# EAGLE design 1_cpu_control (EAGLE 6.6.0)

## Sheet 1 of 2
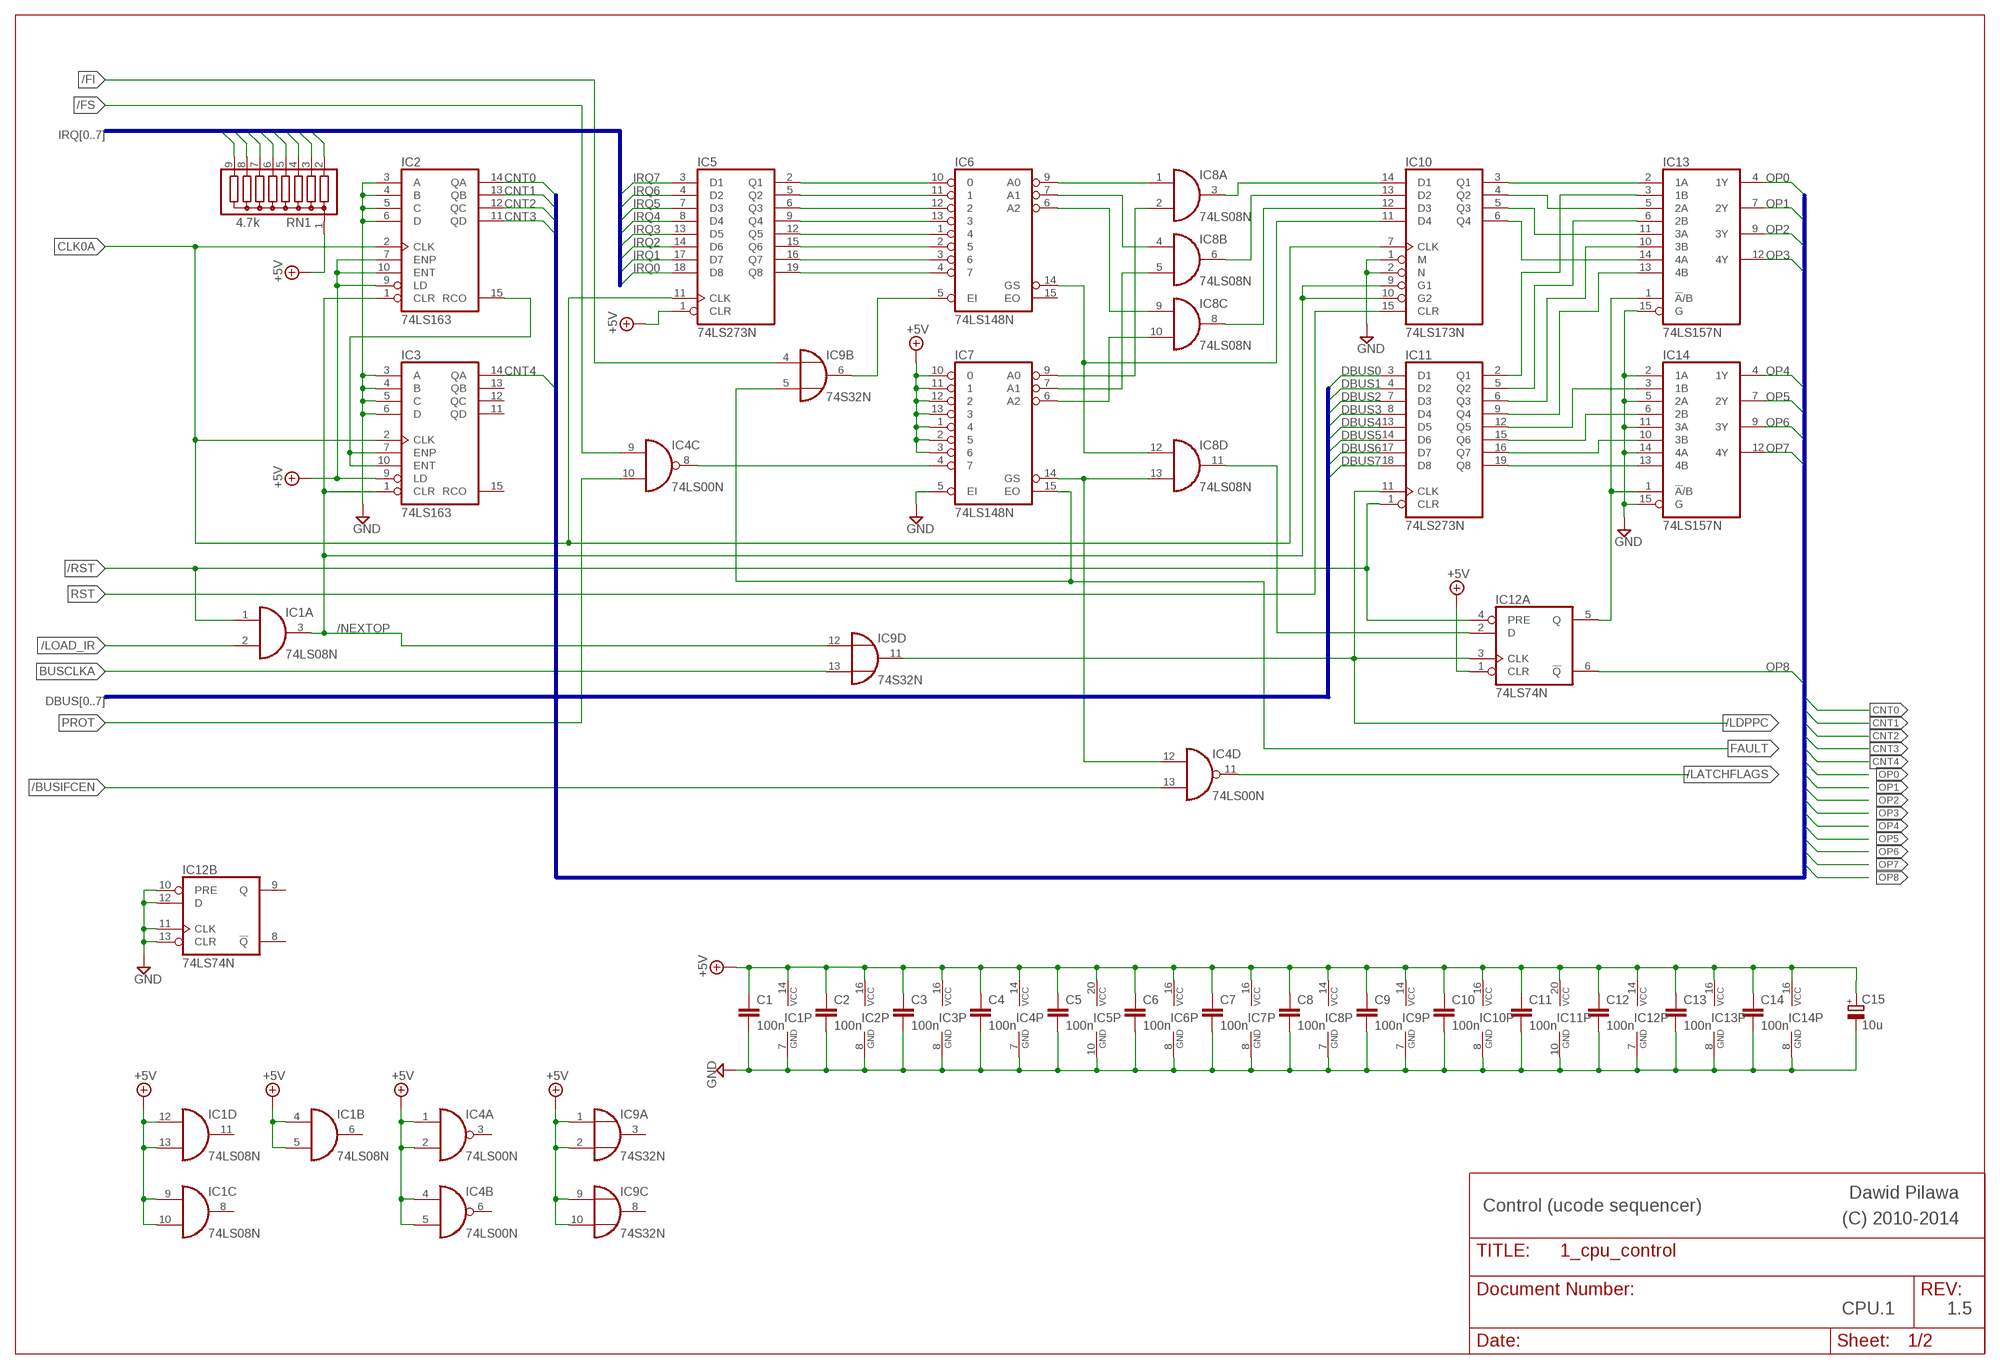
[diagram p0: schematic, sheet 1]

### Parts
C1  100n  C-EU050-024X044  [C050-024X044]
C2  100n  C-EU050-024X044  [C050-024X044]
C3  100n  C-EU050-024X044  [C050-024X044]
C4  100n  C-EU050-024X044  [C050-024X044]
C5  100n  C-EU050-024X044  [C050-024X044]
C6  100n  C-EU050-024X044  [C050-024X044]
C7  100n  C-EU050-024X044  [C050-024X044]
C8  100n  C-EU050-024X044  [C050-024X044]
C9  100n  C-EU050-024X044  [C050-024X044]
C10  100n  C-EU050-024X044  [C050-024X044]
C11  100n  C-EU050-024X044  [C050-024X044]
C12  100n  C-EU050-024X044  [C050-024X044]
C13  100n  C-EU050-024X044  [C050-024X044]
C14  100n  C-EU050-024X044  [C050-024X044]
C15  10u  CPOL-EUE5-6  [E5-6]
IC1  74LS08N  [DIL14]
IC2  74LS163  74160N  [DIL16]
IC3  74LS163  74160N  [DIL16]
IC4  74LS00N  [DIL14]
IC5  74LS273N  74273N  [DIL20]
IC6  74LS148N  [DIL16]
IC7  74LS148N  [DIL16]
IC8  74LS08N  [DIL14]
IC9  74S32N  [DIL14]
IC10  74LS173N  [DIL16]
IC11  74LS273N  74273N  [DIL20]
IC12  74LS74N  [DIL14]
IC13  74LS157N  [DIL16]
IC14  74LS157N  [DIL16]
RN1  4.7k  G08R  [SIL9]

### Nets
+5V: C1.1 C2.1 C3.1 C4.1 C5.1 C6.1 C7.1 C8.1 C9.1 C10.1 C11.1 C12.1 C13.1 C14.1 C15.+ IC1.4(B:I0) IC1.5(B:I1) IC1.9(C:I0) IC1.10(C:I1) IC1.12(D:I0) IC1.13(D:I1) IC1.14(P:VCC) IC2.7(ENP) IC2.9(LD) IC2.10(ENT) IC2.16(VCC) IC3.9(LD) IC3.16(VCC) IC4.1(A:I0) IC4.2(A:I1) IC4.4(B:I0) IC4.5(B:I1) IC4.14(P:VCC) IC5.1(CLR) IC5.20(VCC) IC6.16(VCC) IC7.1 IC7.2 IC7.3 IC7.10 IC7.11 IC7.12 IC7.13 IC7.16(VCC) IC8.14(P:VCC) IC9.1(A:I0) IC9.2(A:I1) IC9.9(C:I0) IC9.10(C:I1) IC9.14(P:VCC) IC10.16(VCC) IC11.20(VCC) IC12.1(A:CLR) IC12.14(P:VCC) IC13.16(VCC) IC14.16(VCC) RN1.1 ; also sheet 2
/BUSIFCEN: IC4.13(D:I1) ; also sheet 2
/FAULT_PF: IC4.8(C:O) IC7.4
/FI: IC9.4(B:I0) ; also sheet 2
/FS: IC4.9(C:I0) ; also sheet 2
/LATCHFLAGS: IC4.11(D:O) ; also sheet 2
/LDPPC: IC9.11(D:O) IC11.11(CLK) IC12.3(A:CLK) ; also sheet 2
/LOAD_IR: IC1.2(A:I1) ; also sheet 2
/NEXTOP: IC1.3(A:O) IC2.1(CLR) IC3.1(CLR) IC9.12(D:I0) IC10.9(G1) IC10.10(G2)
/RST: IC1.1(A:I0) IC11.1(CLR) IC12.4(A:PRE) ; also sheet 2
BUSCLKA: IC9.13(D:I1) ; also sheet 2
CLK0A: IC2.2(CLK) IC3.2(CLK) IC5.11(CLK) IC10.7(CLK) ; also sheet 2
CNT0: IC2.14(QA) ; also sheet 2
CNT1: IC2.13(QB) ; also sheet 2
CNT2: IC2.12(QC) ; also sheet 2
CNT3: IC2.11(QD) ; also sheet 2
CNT4: IC3.14(QA) ; also sheet 2
DBUS0: IC11.3(D1) ; also sheet 2
DBUS1: IC11.4(D2) ; also sheet 2
DBUS2: IC11.7(D3) ; also sheet 2
DBUS3: IC11.8(D4) ; also sheet 2
DBUS4: IC11.13(D5) ; also sheet 2
DBUS5: IC11.14(D6) ; also sheet 2
DBUS6: IC11.17(D7) ; also sheet 2
DBUS7: IC11.18(D8) ; also sheet 2
FAULT: IC7.15(EO) IC9.5(B:I1) ; also sheet 2
GND: C1.2 C2.2 C3.2 C4.2 C5.2 C6.2 C7.2 C8.2 C9.2 C10.2 C11.2 C12.2 C13.2 C14.2 C15.- IC1.7(P:GND) IC2.3(A) IC2.4(B) IC2.5(C) IC2.6(D) IC2.8(GND) IC3.3(A) IC3.4(B) IC3.5(C) IC3.6(D) IC3.8(GND) IC4.7(P:GND) IC5.10(GND) IC6.8(GND) IC7.5(EI) IC7.8(GND) IC8.7(P:GND) IC9.7(P:GND) IC10.1(M) IC10.2(N) IC10.8(GND) IC11.10(GND) IC12.7(P:GND) IC12.10(B:PRE) IC12.11(B:CLK) IC12.12(B:D) IC12.13(B:CLR) IC13.8(GND) IC13.15(G) IC14.2(1A) IC14.5(2A) IC14.8(GND) IC14.11(3A) IC14.14(4A) IC14.15(G) ; also sheet 2
IRQ0: IC5.18(D8) RN1.9 ; also sheet 2
IRQ1: IC5.17(D7) RN1.8 ; also sheet 2
IRQ2: IC5.14(D6) RN1.7 ; also sheet 2
IRQ3: IC5.13(D5) RN1.6 ; also sheet 2
IRQ4: IC5.8(D4) RN1.5 ; also sheet 2
IRQ5: IC5.7(D3) RN1.4 ; also sheet 2
IRQ6: IC5.4(D2) RN1.3 ; also sheet 2
IRQ7: IC5.3(D1) RN1.2 ; also sheet 2
N$1: IC6.9(A0) IC8.1(A:I0)
N$2: IC2.15(RCO) IC3.7(ENP) IC3.10(ENT)
N$3: IC7.9(A0) IC8.2(A:I1)
N$4: IC6.7(A1) IC8.4(B:I0)
N$5: IC7.7(A1) IC8.5(B:I1)
N$6: IC7.6(A2) IC8.10(C:I1)
N$7: IC6.6(A2) IC8.9(C:I0)
N$9: IC6.14(GS) IC8.12(D:I0) IC10.11(D4)
N$10: IC4.12(D:I0) IC7.14(GS) IC8.13(D:I1)
N$11: IC8.3(A:O) IC10.14(D1)
N$12: IC8.6(B:O) IC10.13(D2)
N$13: IC8.8(C:O) IC10.12(D3)
N$14: IC8.11(D:O) IC12.2(A:D)
N$16: IC11.5(Q2) IC13.6(2B)
N$18: IC10.3(Q1) IC13.2(1A)
N$19: IC10.4(Q2) IC13.5(2A)
N$20: IC10.5(Q3) IC13.11(3A)
N$21: IC10.6(Q4) IC13.14(4A)
N$22: IC11.19(Q8) IC14.13(4B)
N$23: IC11.16(Q7) IC14.10(3B)
N$24: IC11.15(Q6) IC14.6(2B)
N$25: IC11.12(Q5) IC14.3(1B)
N$26: IC11.2(Q1) IC13.3(1B)
N$27: IC6.5(EI) IC9.6(B:O)
N$28: IC11.6(Q3) IC13.10(3B)
N$30: IC11.9(Q4) IC13.13(4B)
N$47: IC12.5(A:Q) IC13.1(!A!/B) IC14.1(!A!/B)
N$57: IC5.19(Q8) IC6.4
N$58: IC5.16(Q7) IC6.3
N$59: IC5.15(Q6) IC6.2
N$60: IC5.12(Q5) IC6.1
N$61: IC5.9(Q4) IC6.13
N$62: IC5.6(Q3) IC6.12
N$63: IC5.5(Q2) IC6.11
N$64: IC5.2(Q1) IC6.10
OP0: IC13.4(1Y) ; also sheet 2
OP1: IC13.7(2Y) ; also sheet 2
OP2: IC13.9(3Y) ; also sheet 2
OP3: IC13.12(4Y) ; also sheet 2
OP4: IC14.4(1Y) ; also sheet 2
OP5: IC14.7(2Y) ; also sheet 2
OP6: IC14.9(3Y) ; also sheet 2
OP7: IC14.12(4Y) ; also sheet 2
OP8: IC12.6(A:!Q) ; also sheet 2
PROT: IC4.10(C:I1) ; also sheet 2
RST: IC10.15(CLR) ; also sheet 2
Unconnected: IC1.6(B:O) IC1.8(C:O) IC1.11(D:O) IC3.11(QD) IC3.12(QC) IC3.13(QB) IC3.15(RCO) IC4.3(A:O) IC4.6(B:O) IC6.15(EO) IC9.3(A:O) IC9.8(C:O) IC12.8(B:!Q) IC12.9(B:Q)

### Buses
DBUS[0..7]
UCADR:OP[0..8],CNT[0..4]
IRQ[0..7]

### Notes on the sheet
- Dawid Pilawa
- Control (ucode sequencer) | (C) 2010-2014
- CPU.1 | 1.5

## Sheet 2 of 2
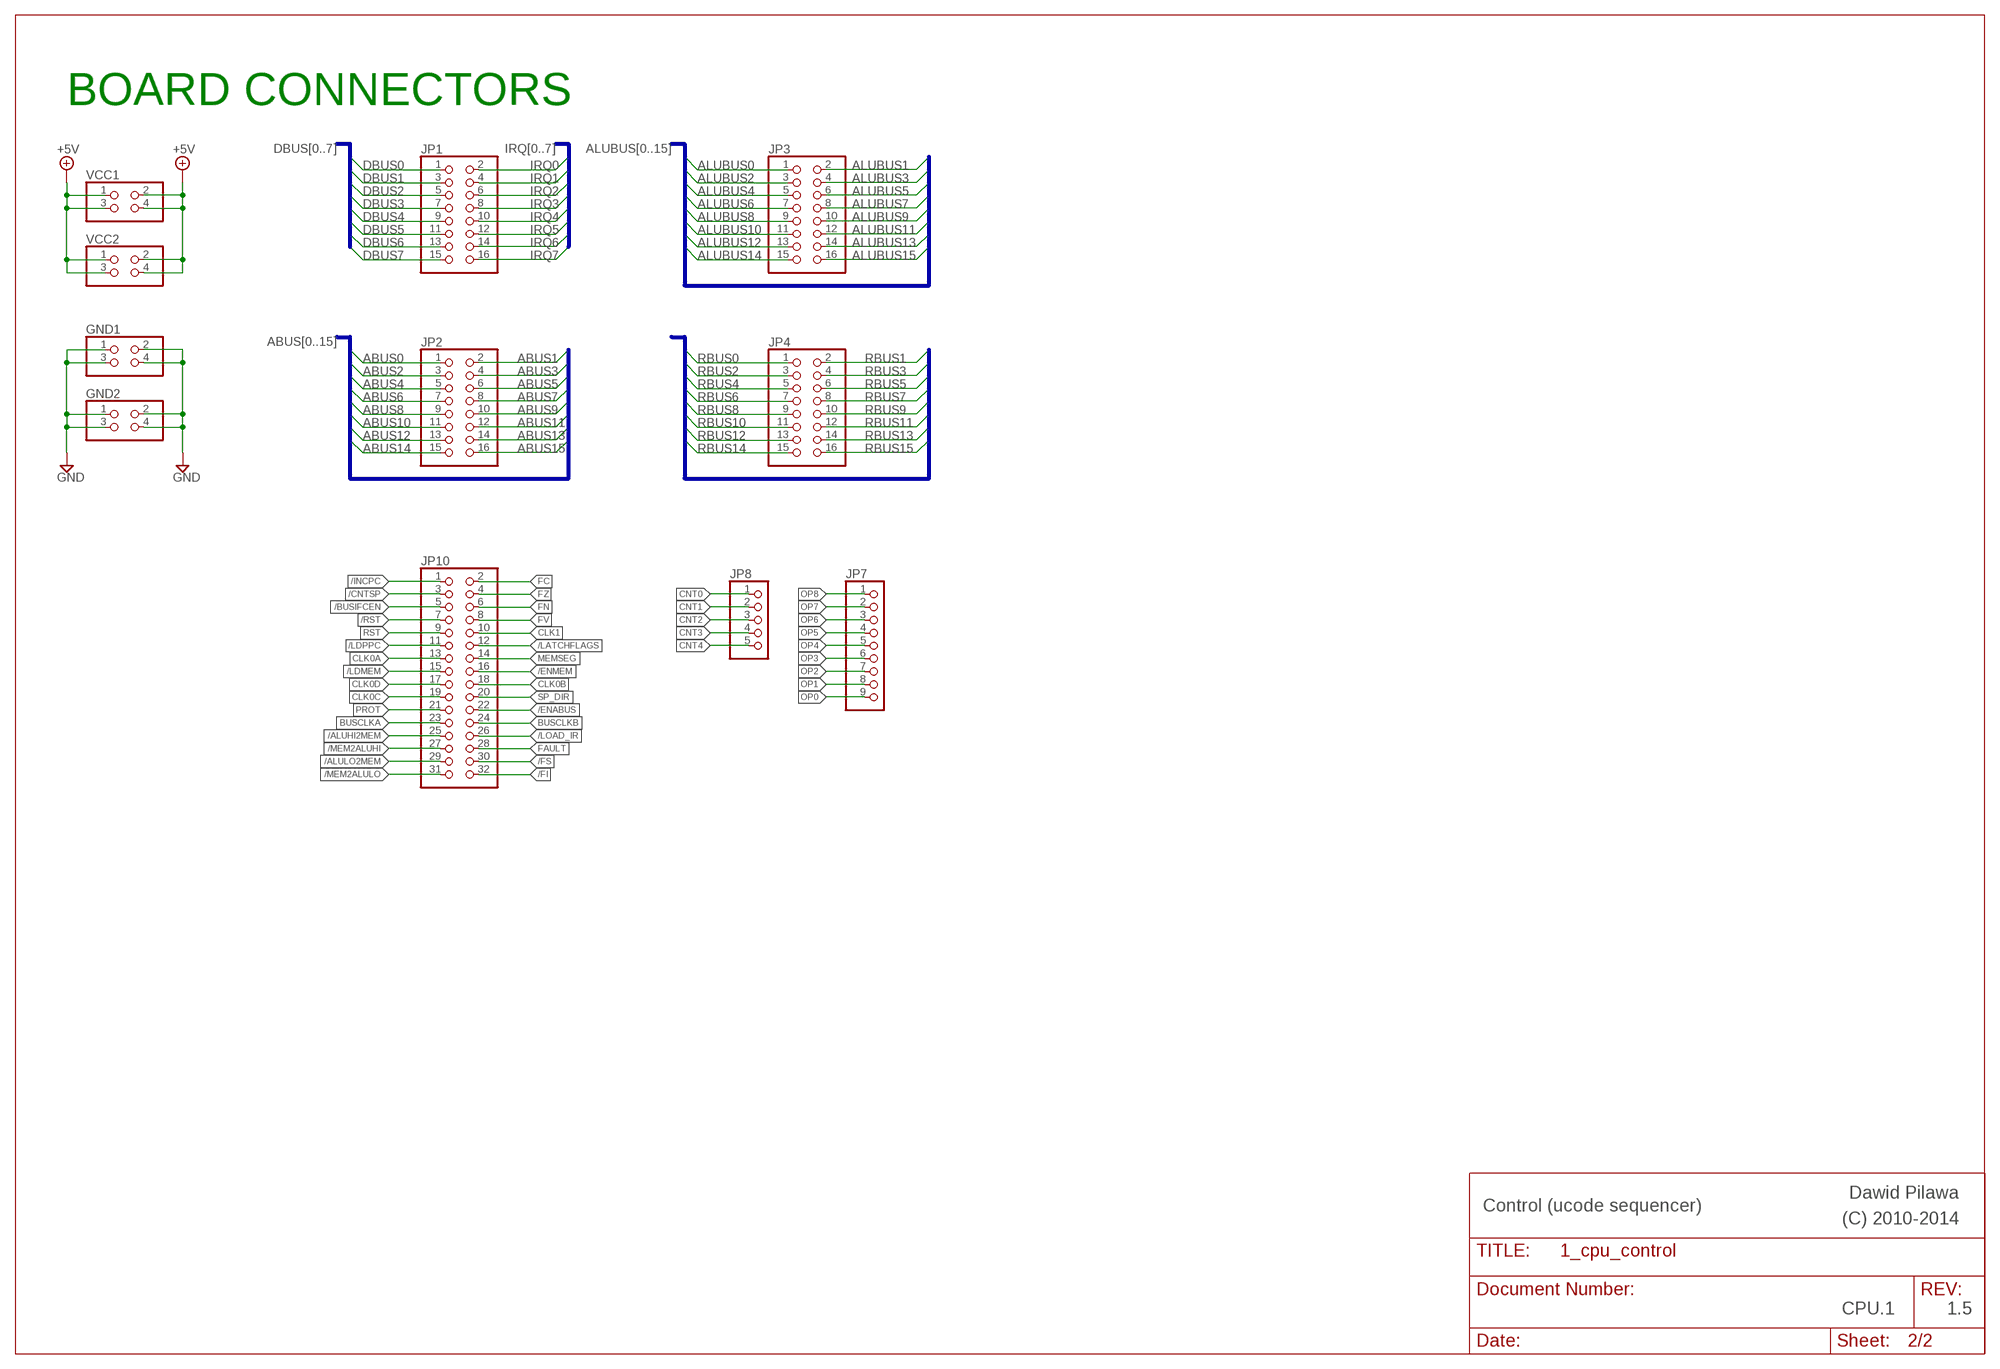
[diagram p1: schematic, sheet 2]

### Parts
GND1  PINHD-2X2  [2X02]
GND2  PINHD-2X2  [2X02]
JP1  PINHD-2X8  [2X08]
JP2  PINHD-2X8  [2X08]
JP3  PINHD-2X8  [2X08]
JP4  PINHD-2X8  [2X08]
JP7  PINHD-1X9  [1X09]
JP8  PINHD-1X5  [1X05]
JP10  PINHD-2X16  [2X16]
VCC1  PINHD-2X2  [2X02]
VCC2  PINHD-2X2  [2X02]

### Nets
+5V: VCC1.1 VCC1.2 VCC1.3 VCC1.4 VCC2.1 VCC2.2 VCC2.3 VCC2.4 ; also sheet 1
/ALUHI2MEM: JP10.25
/ALULO2MEM: JP10.29
/BUSIFCEN: JP10.5 ; also sheet 1
/CNTSP: JP10.3
/ENABUS: JP10.22
/ENMEM: JP10.16
/FI: JP10.32 ; also sheet 1
/FS: JP10.30 ; also sheet 1
/INCPC: JP10.1
/LATCHFLAGS: JP10.12 ; also sheet 1
/LDMEM: JP10.15
/LDPPC: JP10.11 ; also sheet 1
/LOAD_IR: JP10.26 ; also sheet 1
/MEM2ALUHI: JP10.27
/MEM2ALULO: JP10.31
/RST: JP10.7 ; also sheet 1
ABUS0: JP2.1
ABUS1: JP2.2
ABUS2: JP2.3
ABUS3: JP2.4
ABUS4: JP2.5
ABUS5: JP2.6
ABUS6: JP2.7
ABUS7: JP2.8
ABUS8: JP2.9
ABUS9: JP2.10
ABUS10: JP2.11
ABUS11: JP2.12
ABUS12: JP2.13
ABUS13: JP2.14
ABUS14: JP2.15
ABUS15: JP2.16
ALUBUS0: JP3.1
ALUBUS1: JP3.2
ALUBUS2: JP3.3
ALUBUS3: JP3.4
ALUBUS4: JP3.5
ALUBUS5: JP3.6
ALUBUS6: JP3.7
ALUBUS7: JP3.8
ALUBUS8: JP3.9
ALUBUS9: JP3.10
ALUBUS10: JP3.11
ALUBUS11: JP3.12
ALUBUS12: JP3.13
ALUBUS13: JP3.14
ALUBUS14: JP3.15
ALUBUS15: JP3.16
BUSCLKA: JP10.23 ; also sheet 1
BUSCLKB: JP10.24
CLK0A: JP10.13 ; also sheet 1
CLK0B: JP10.18
CLK0C: JP10.19
CLK0D: JP10.17
CLK1: JP10.10
CNT0: JP8.1 ; also sheet 1
CNT1: JP8.2 ; also sheet 1
CNT2: JP8.3 ; also sheet 1
CNT3: JP8.4 ; also sheet 1
CNT4: JP8.5 ; also sheet 1
DBUS0: JP1.1 ; also sheet 1
DBUS1: JP1.3 ; also sheet 1
DBUS2: JP1.5 ; also sheet 1
DBUS3: JP1.7 ; also sheet 1
DBUS4: JP1.9 ; also sheet 1
DBUS5: JP1.11 ; also sheet 1
DBUS6: JP1.13 ; also sheet 1
DBUS7: JP1.15 ; also sheet 1
FAULT: JP10.28 ; also sheet 1
FC: JP10.2
FN: JP10.6
FV: JP10.8
FZ: JP10.4
GND: GND1.1 GND1.2 GND1.3 GND1.4 GND2.1 GND2.2 GND2.3 GND2.4 ; also sheet 1
IRQ0: JP1.2 ; also sheet 1
IRQ1: JP1.4 ; also sheet 1
IRQ2: JP1.6 ; also sheet 1
IRQ3: JP1.8 ; also sheet 1
IRQ4: JP1.10 ; also sheet 1
IRQ5: JP1.12 ; also sheet 1
IRQ6: JP1.14 ; also sheet 1
IRQ7: JP1.16 ; also sheet 1
MEMSEG: JP10.14
OP0: JP7.9 ; also sheet 1
OP1: JP7.8 ; also sheet 1
OP2: JP7.7 ; also sheet 1
OP3: JP7.6 ; also sheet 1
OP4: JP7.5 ; also sheet 1
OP5: JP7.4 ; also sheet 1
OP6: JP7.3 ; also sheet 1
OP7: JP7.2 ; also sheet 1
OP8: JP7.1 ; also sheet 1
PROT: JP10.21 ; also sheet 1
RBUS0: JP4.1
RBUS1: JP4.2
RBUS2: JP4.3
RBUS3: JP4.4
RBUS4: JP4.5
RBUS5: JP4.6
RBUS6: JP4.7
RBUS7: JP4.8
RBUS8: JP4.9
RBUS9: JP4.10
RBUS10: JP4.11
RBUS11: JP4.12
RBUS12: JP4.13
RBUS13: JP4.14
RBUS14: JP4.15
RBUS15: JP4.16
RST: JP10.9 ; also sheet 1
SP_DIR: JP10.20

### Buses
DBUS[0..7]
IRQ[0..7]
ALUBUS[0..15]
RBUS[0..15]
ABUS[0..15]

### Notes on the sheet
- BOARD CONNECTORS
- Dawid Pilawa
- Control (ucode sequencer) | (C) 2010-2014
- CPU.1 | 1.5

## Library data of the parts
C1-C14 = rcl:C-EU: CAPACITOR, European symbol
C15 = rcl:CPOL-EU: POLARIZED CAPACITOR, European symbol
GND1 GND2 VCC1 VCC2 = pinhead:PINHD-2X2: PIN HEADER
IC1 IC8 = 74xx-eu:74*08: Quad 2-input AND gate
IC2 IC3 = 74xx-eu:74*160: Synchronous 4-bit COUNTER
IC4 = 74xx-eu:74*00: Quad 2-input NAND gate
IC5 IC11 = 74xx-eu:74*273: Octal D type FLIP FLOP, clear
IC6 IC7 = 74xx-eu:74*148: 10-line to 4-line and 8-line to 3-line PRIORITY ENCODER
IC9 = 74xx-eu:74*32: Quad 2-input OR gate
IC10 = 74xx-eu:74*173: 4-bit D type REGISTER, 3-state
IC12 = 74xx-eu:74*74: Dual D type positive edge triggered FLIP FLOP, preset and clear
IC13 IC14 = 74xx-eu:74*157: Quadruple 2-line to 1-line data SELECTOR/MULTIPLEXER
JP1-JP4 = pinhead:PINHD-2X8: PIN HEADER
JP7 = pinhead:PINHD-1X9: PIN HEADER
JP8 = pinhead:PINHD-1X5: PIN HEADER
JP10 = pinhead:PINHD-2X16: PIN HEADER
RN1 = resistor-sil:G08R: SIL RESISTOR

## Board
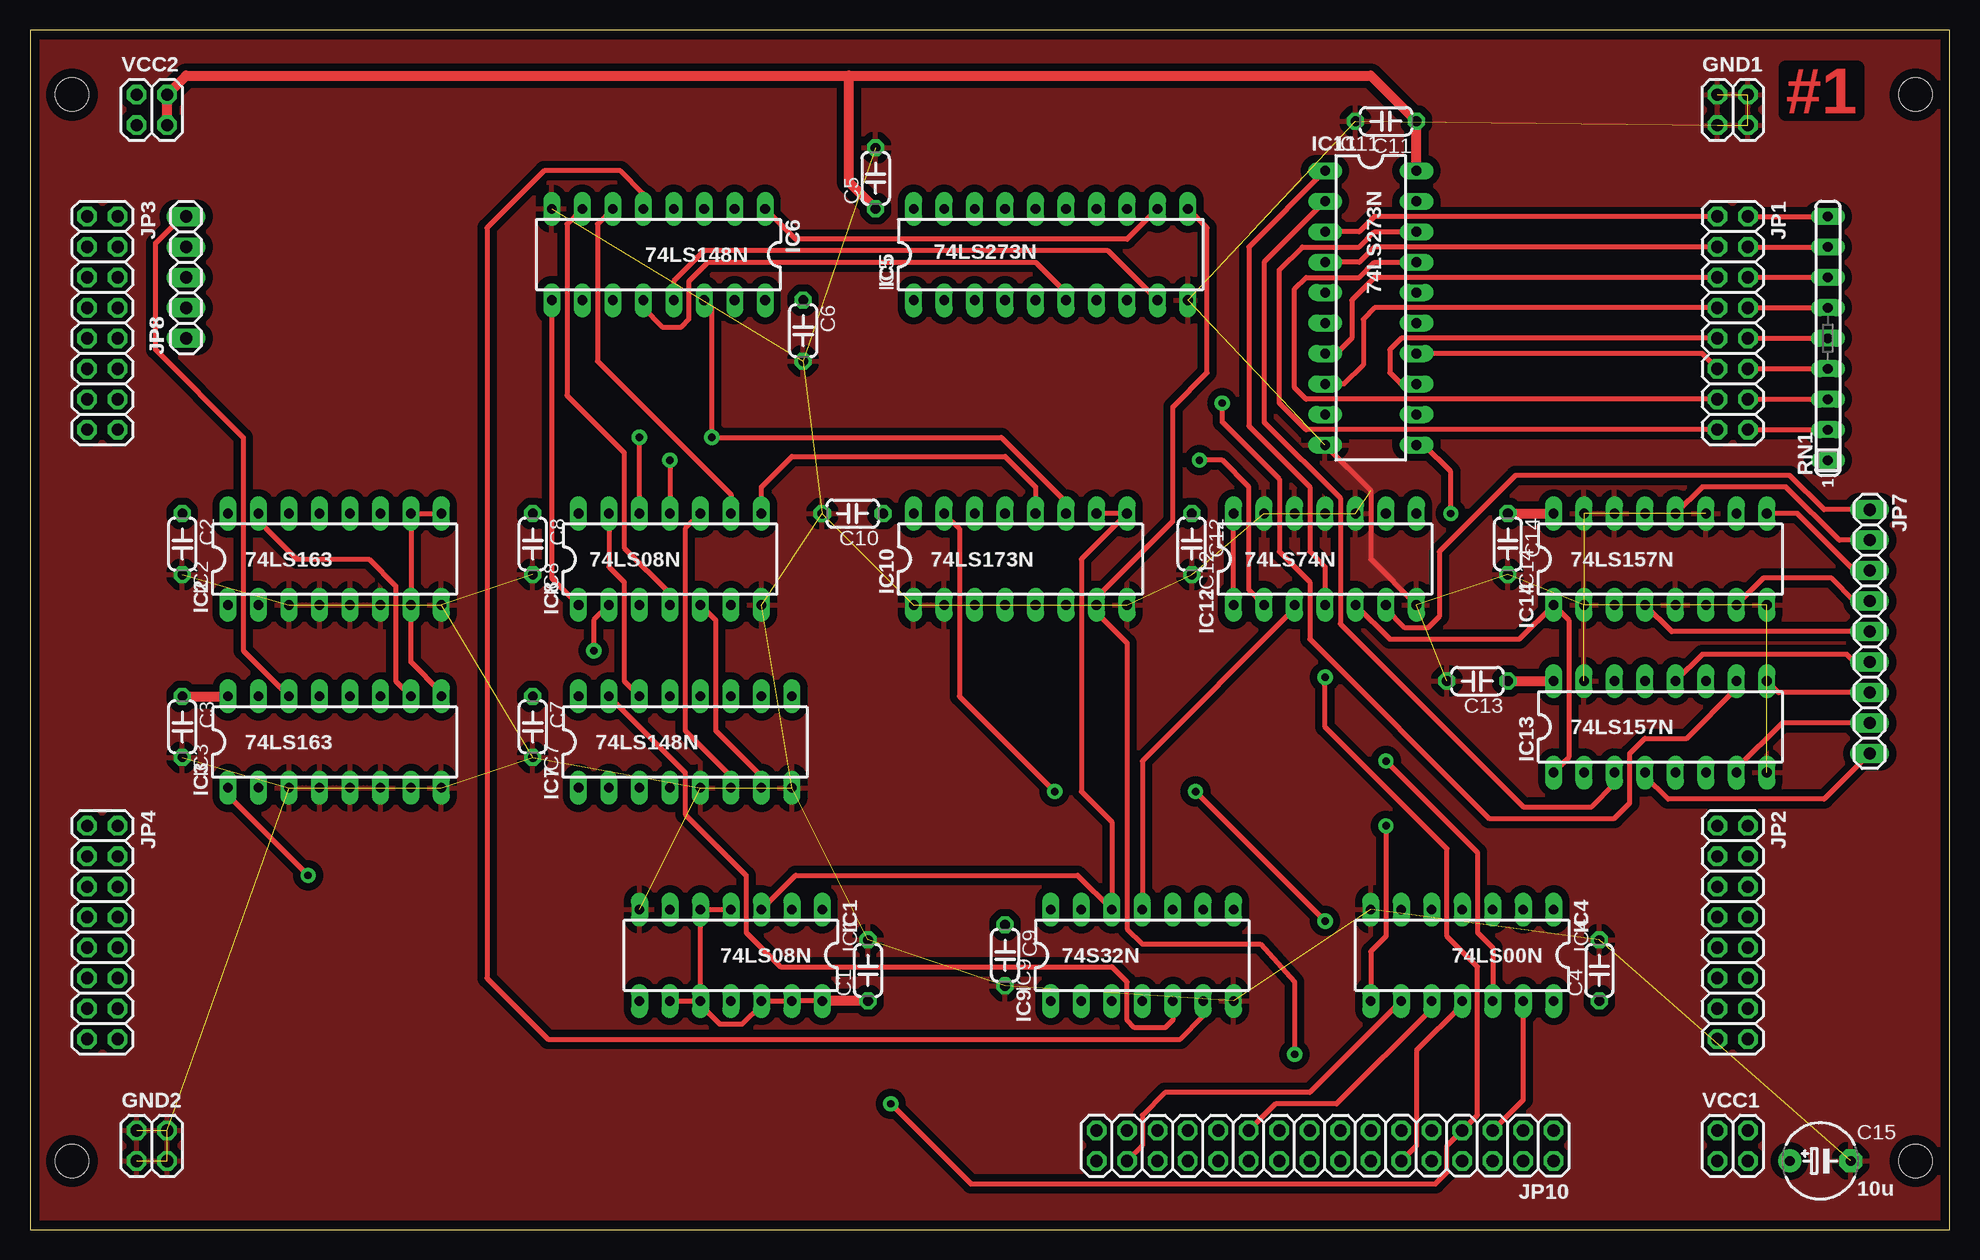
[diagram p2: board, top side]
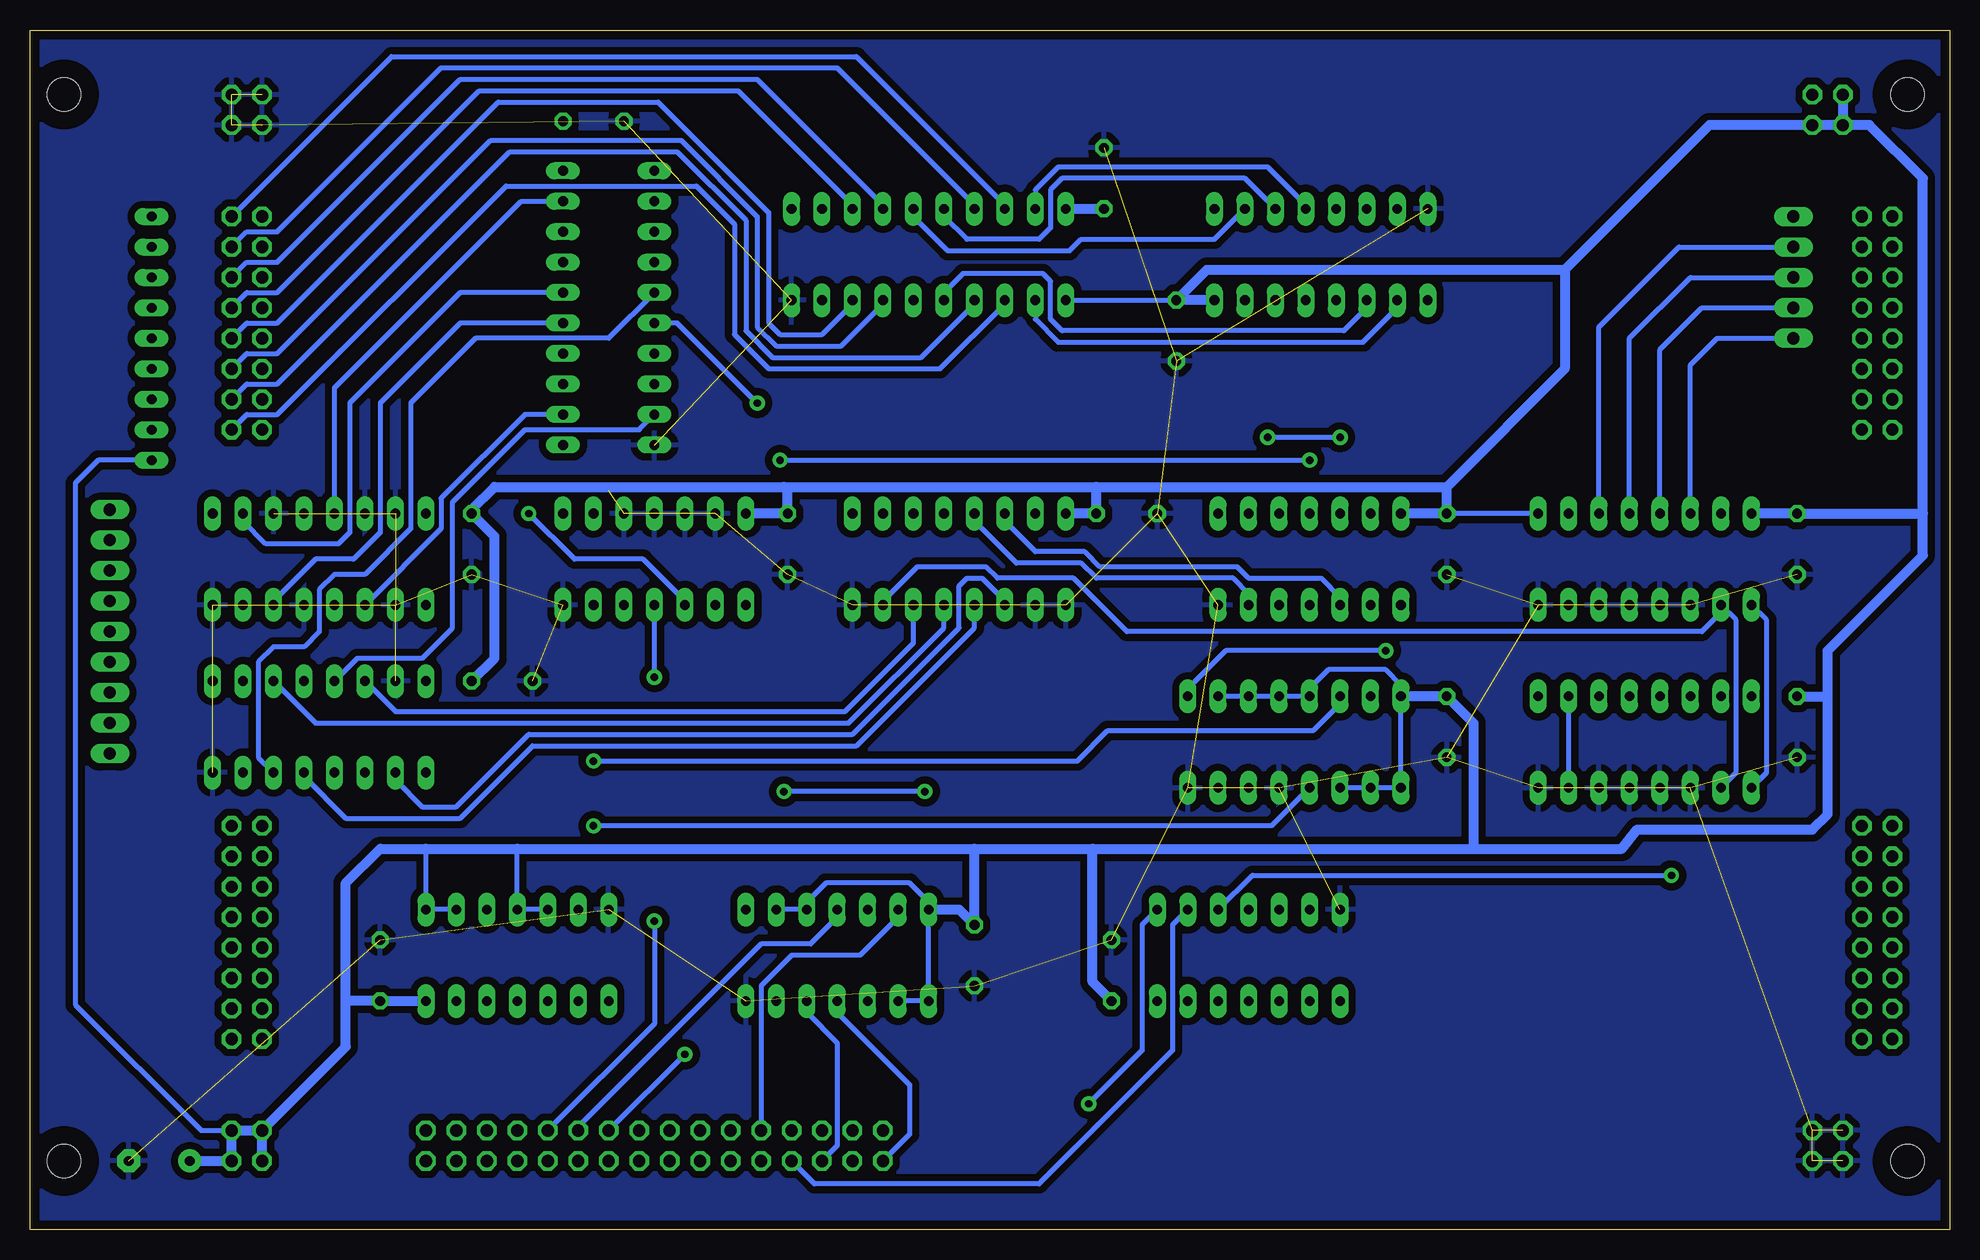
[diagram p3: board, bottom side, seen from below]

Size 160 x 100 mm. Coordinates in mm from the lower left corner, seen from the top.
Outline: 0,0 160,0 160,100 0,100 0,0
Copper layers (1*16): Top 0.035mm / dielectric 1.5mm / Bottom 0.035mm
Design rules "homebrew_pcb": minimum track width 16mil, minimum drill 24mil, track to track 16mil, track to pad 10mil, pad to pad 10mil, via to via 10mil, smd to smd 8mil, copper to edge 30mil, drill to drill 10mil, minimum pad ring 12mil, minimum via ring 12mil, stop-mask expansion 4mil, vias tented up to drill 0mil, thermal gap 24mil
Holes 2.79 mm at 3.49,94.61 3.49,5.71 157.16,94.61 157.16,5.71
bRestrict: area 1.2,92.3 to 5.8,96.9; area 154.9,92.3 to 159.4,96.9; area 154.9,3.4 to 159.4,8; area 1.2,3.4 to 5.8,8
vRestrict: area 1.2,92.3 to 5.8,96.9; area 1.2,3.4 to 5.8,8; area 154.9,3.4 to 159.4,8; area 154.9,92.3 to 159.4,96.9

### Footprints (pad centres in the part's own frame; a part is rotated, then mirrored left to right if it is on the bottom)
C050-024X044 = drill 0.813 octagon: 1 -2.54,0; 2 2.54,0
E5-6 = drill 0.813 pad 1.905: + -2.54,0 | drill 0.813 pad 1.905 octagon: - 2.54,0
2X02 = drill 1.016 octagon: 1 -1.27,-1.27; 2 -1.27,1.27; 3 1.27,-1.27; 4 1.27,1.27
DIL14 = drill 0.813 long: 1 -7.62,-3.81; 2 -5.08,-3.81; 3 -2.54,-3.81; 4 0,-3.81; 5 2.54,-3.81; 6 5.08,-3.81; 7 7.62,-3.81; 8 7.62,3.81; 9 5.08,3.81; 10 2.54,3.81; 11 0,3.81; 12 -2.54,3.81; 13 -5.08,3.81; 14 -7.62,3.81
DIL16 = drill 0.813 long: 1 -8.89,-3.81; 2 -6.35,-3.81; 3 -3.81,-3.81; 4 -1.27,-3.81; 5 1.27,-3.81; 6 3.81,-3.81; 7 6.35,-3.81; 8 8.89,-3.81; 9 8.89,3.81; 10 6.35,3.81; 11 3.81,3.81; 12 1.27,3.81; 13 -1.27,3.81; 14 -3.81,3.81; 15 -6.35,3.81; 16 -8.89,3.81
DIL20 = drill 0.813 long: 1 -11.43,-3.81; 2 -8.89,-3.81; 3 -6.35,-3.81; 4 -3.81,-3.81; 5 -1.27,-3.81; 6 1.27,-3.81; 7 3.81,-3.81; 8 6.35,-3.81; 9 8.89,-3.81; 10 11.43,-3.81; 11 11.43,3.81; 12 8.89,3.81; 13 6.35,3.81; 14 3.81,3.81; 15 1.27,3.81; 16 -1.27,3.81; 17 -3.81,3.81; 18 -6.35,3.81; 19 -8.89,3.81; 20 -11.43,3.81
2X08 = drill 1.016 octagon: 1 -8.89,-1.27; 2 -8.89,1.27; 3 -6.35,-1.27; 4 -6.35,1.27; 5 -3.81,-1.27; 6 -3.81,1.27; 7 -1.27,-1.27; 8 -1.27,1.27; 9 1.27,-1.27; 10 1.27,1.27; 11 3.81,-1.27; 12 3.81,1.27; 13 6.35,-1.27; 14 6.35,1.27; 15 8.89,-1.27; 16 8.89,1.27
1X09 = drill 1.016 long: 1 -10.16,0; 2 -7.62,0; 3 -5.08,0; 4 -2.54,0; 5 0,0; 6 2.54,0; 7 5.08,0; 8 7.62,0; 9 10.16,0
1X05 = drill 1.016 long: 1 -5.08,0; 2 -2.54,0; 3 0,0; 4 2.54,0; 5 5.08,0
2X16 = drill 1.016 octagon: 1 -19.05,-1.27; 2 -19.05,1.27; 3 -16.51,-1.27; 4 -16.51,1.27; 5 -13.97,-1.27; 6 -13.97,1.27; 7 -11.43,-1.27; 8 -11.43,1.27; 9 -8.89,-1.27; 10 -8.89,1.27; 11 -6.35,-1.27; 12 -6.35,1.27; 13 -3.81,-1.27; 14 -3.81,1.27; 15 -1.27,-1.27; 16 -1.27,1.27; 17 1.27,-1.27; 18 1.27,1.27; 19 3.81,-1.27; 20 3.81,1.27; 21 6.35,-1.27; 22 6.35,1.27; 23 8.89,-1.27; 24 8.89,1.27; 25 11.43,-1.27; 26 11.43,1.27; 27 13.97,-1.27; 28 13.97,1.27; 29 16.51,-1.27; 30 16.51,1.27; 31 19.05,-1.27; 32 19.05,1.27
SIL9 = drill 0.813 long: 1 -10.16,0; 2 -7.62,0; 3 -5.08,0; 4 -2.54,0; 5 0,0; 6 2.54,0; 7 5.08,0; 8 7.62,0; 9 10.16,0

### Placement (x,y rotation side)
C1  69.85,21.59 90 top
C2  12.7,57.15 270 top
C3  12.7,41.91 270 top
C4  130.81,21.59 90 top
C5  70.48,87.63 90 top
C6  64.45,74.93 270 top
C7  41.91,41.91 270 top
C8  41.91,57.15 270 top
C9  81.28,22.86 270 top
C10  68.58,59.69 180 top
C11  113.03,92.39 180 top
C12  96.84,57.15 270 top
C13  120.65,45.72 180 top
C14  123.19,57.15 270 top
C15  149.22,5.71 0 top
GND1  141.92,93.34 0 top
GND2  10.16,6.99 0 top
IC1  58.42,22.86 180 top
IC2  25.4,55.88 0 top
IC3  25.4,40.64 0 top
IC4  119.38,22.86 180 top
IC5  85.09,81.28 0 top
IC6  52.39,81.28 180 top
IC7  54.61,40.64 0 top
IC8  53.34,55.88 0 top
IC9  92.71,22.86 0 top
IC10  82.55,55.88 0 top
IC11  111.76,76.83 270 top
IC12  107.95,55.88 0 top
IC13  135.89,41.91 0 top
IC14  135.89,55.88 0 top
JP1  141.92,75.56 270 top
JP2  141.92,24.77 270 top
JP3  6.03,75.56 270 top
JP4  6.03,24.77 270 top
JP7  153.35,49.85 270 top
JP8  13.02,79.38 90 top
JP10  107.95,6.99 180 top
RN1  149.86,74.3 90 top
VCC1  141.92,6.99 0 top
VCC2  10.16,93.34 0 top

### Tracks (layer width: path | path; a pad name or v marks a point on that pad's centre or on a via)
+5V
  Top 0.406: IC2.9 IC2.10 IC2.7 31.75,47.31 34.29,44.77 IC3.9 | IC1.10 IC1.5 IC1.4 | IC1.9 IC1.10 | IC1.14 IC1.13 IC1.12 60.96,18.73 59.37,17.14 57.47,17.14 55.88,18.73 IC1.10 | IC12.1 IC12.14
  Top 0.813: 68.26,96.2 13.02,96.2 VCC2.4 VCC2.3 | 68.26,96.2 111.76,96.2 C11.1 IC11.20 | C1.1 IC1.14 | C3.1 IC3.16 | C14.1 IC14.16 | C13.1 IC13.16 | C5.1 68.26,87.31 68.26,96.2
  Bottom 0.406: RN1.1 154.31,64.14 156.21,62.23 156.21,18.73 145.73,8.26 VCC1.4 | IC2.9 C8.1 | 127,31.75 IC4.1 IC4.2 | IC4.5 IC4.4 119.38,31.75 | IC5.1 C6.1 | IC7.3 IC7.2 IC7.1 IC7.16 45.72,45.4 46.99,46.67 51.75,46.67 53.34,45.09 IC7.13 IC7.12 IC7.11 IC7.10 | IC9.9 IC9.10 95.25,27.3 93.66,28.89 86.68,28.89 85.09,27.3 IC9.14 IC9.1 IC9.2
  Bottom 0.813: VCC1.2 133.67,15.24 133.67,19.05 | 133.67,19.05 133.67,28.89 130.81,31.75 127,31.75 119.38,31.75 81.28,31.75 | 81.28,31.75 71.44,31.75 | 71.44,31.75 39.69,31.75 | 39.69,31.75 27.3,31.75 26.04,33.34 11.43,33.34 10.16,34.61 10.16,44.45 | 10.16,44.45 10.16,48.26 2.22,56.2 2.22,59.69 | 2.22,59.69 2.22,87.63 6.67,92.08 VCC2.1 | VCC2.1 VCC2.3 20,92.08 32.07,80.01 | VCC2.2 VCC2.1 | VCC1.1 VCC1.2 | VCC1.2 VCC1.4 VCC1.3 C15.+ | 133.67,19.05 C4.1 IC4.14 | 81.28,31.75 C9.1 82.55,26.67 IC9.14 | C1.1 71.44,20.64 71.44,31.75 | C3.1 10.16,44.45 | 2.22,59.69 C2.1 IC2.16 | 39.69,31.75 39.69,42.23 C7.1 IC7.16 | 97.16,61.91 121.28,61.91 123.19,60.01 C14.1 121.28,57.78 121.28,47.62 C13.1 | 97.16,61.91 71.12,61.91 | 71.12,61.91 41.91,61.91 | 32.07,80.01 32.07,71.75 41.91,61.91 | 41.91,61.91 C8.1 IC8.14 | 71.12,61.91 C10.1 IC10.16 | 97.16,61.91 96.84,61.59 C12.1 IC12.14 | IC5.20 C5.1 | 32.07,80.01 61.91,80.01 C6.1 IC6.16
/BUSIFCEN
  Top 0.406: JP10.5 124.46,10.79 IC4.13
/FAULT_PF  (via drill 0.61 pad 1.27)
  Top 0.406: v113.03,33.66 113.03,24.45 111.76,23.18 IC4.8
  Bottom 0.406: IC7.4 56.52,33.66 v113.03,33.66
/FI
  Bottom 0.406: IC9.4 92.71,18.1 86.68,12.06 86.68,7.94 JP10.32
/FS
  Top 0.406: IC4.9 106.68,11.43 94.61,11.43 92.71,9.53 92.71,6.99 JP10.30
/LATCHFLAGS
  Top 0.406: JP10.12 115.57,6.99 115.57,14.92 119.38,18.73 IC4.11
/LDPPC  (via drill 0.61 pad 1.27)
  Top 0.406: v118.43,59.69 118.43,63.18 116.2,65.41 IC11.11 | IC9.11 92.71,39.05 105.41,51.75 IC12.3
  Bottom 0.406: v118.43,59.69 114.62,55.88 108.9,55.88 105.41,52.39 IC12.3 | IC9.11 92.71,26.04 94.93,23.81 99.06,23.81 114.3,8.57 JP10.11
/LOAD_IR
  Bottom 0.406: IC1.2 64.77,25.4 64.77,14.92 75.88,3.81 94.61,3.81 JP10.26
/NEXTOP  (via drill 0.61 pad 1.27)
  Top 0.406: v23.18,29.53 16.51,36.2 IC3.1 | IC10.10 IC10.9 87.63,55.88 87.63,36.51 90.17,33.97 IC9.12 87.31,29.53 63.82,29.53 IC1.3
  Bottom 0.406: IC3.1 15.24,38.1 15.24,50.8 IC2.1 | IC1.3 58.1,29.53 v23.18,29.53
/RST  (via drill 0.61 pad 1.27)
  Top 0.406: IC11.1 101.6,81.92 101.6,66.99 106.68,61.91 106.68,56.52 107.95,55.24 IC12.4 | v71.75,10.48 78.42,3.81 117.16,3.81 118.11,4.76 118.11,6.99 JP10.7 120.65,9.53 120.65,21.91 118.11,24.45 118.11,31.75 107.95,41.91 v107.95,46.04
  Bottom 0.406: v107.95,46.04 IC12.4 | IC1.1 67.31,25.4 67.31,14.92 v71.75,10.48
BUSCLKA
  Bottom 0.406: IC9.13 87.63,26.04 90.81,22.86 96.52,22.86 99.06,20.32 JP10.23
CLK0A  (via drill 0.61 pad 1.27)
  Top 0.406: v105.41,14.61 105.41,20.64 102.55,23.81 92.71,23.81 91.44,25.08 91.44,48.9 88.9,51.44 IC10.7 88.9,52.7 95.25,59.05 95.25,68.58 98.11,71.44 98.11,83.5 IC5.11
  Bottom 0.406: IC3.2 17.78,38.1 17.78,50.8 IC2.2 19.05,51.44 20.64,49.85 68.58,49.85 73.03,54.29 79.38,54.29 80.33,55.24 86.04,55.24 88.9,52.39 IC10.7 | v105.41,14.61 JP10.13
CNT0
  Bottom 0.406: IC2.14 21.59,72.07 19.37,74.3 JP8.1
CNT1
  Bottom 0.406: IC2.13 24.13,73.34 20.64,76.83 JP8.2
CNT2
  Bottom 0.406: IC2.12 26.67,74.3 21.59,79.38 JP8.3
CNT3
  Bottom 0.406: IC2.11 29.21,75.25 22.54,81.92 JP8.4
CNT4
  Top 0.406: IC3.14 20.8,45.24 20.32,45.72 17.78,48.26 17.78,66.04 10.48,73.34 10.48,82.23 12.7,84.45 JP8.5
DBUS0
  Top 0.406: JP1.1 112.08,84.45 110.81,83.19 IC11.3
DBUS1
  Top 0.406: JP1.3 112.08,81.92 110.81,80.64 IC11.4
DBUS2
  Top 0.406: JP1.5 112.08,79.38 110.17,77.47 110.17,74.3 108.9,73.03 IC11.7
DBUS3
  Top 0.406: JP1.7 112.08,76.83 111.12,75.88 111.12,72.07 109.54,70.48 IC11.8
DBUS4
  Top 0.406: JP1.9 114.3,74.3 113.35,73.34 113.35,71.44 114.3,70.48 IC11.13
DBUS5
  Top 0.406: JP1.11 139.38,73.03 IC11.14
DBUS6
  Top 0.406: JP1.13 106.36,69.22 105.41,70.17 105.41,78.42 106.36,79.38 110.81,79.38 112.08,80.64 IC11.17
DBUS7
  Top 0.406: JP1.15 106.36,66.67 104.14,68.9 104.14,80.01 106.05,81.92 110.81,81.92 112.08,83.19 IC11.18
FAULT
  Top 0.406: IC7.15 54.61,38.1 54.61,34.61 59.69,29.53 59.69,24.77 62.55,21.91 90.17,21.91 91.44,20.64 91.44,17.46 92.08,16.83 94.61,16.83 95.25,17.46 IC9.5
  Bottom 0.406: IC9.5 95.25,18.1 92.71,15.56 92.71,6.99 JP10.28
GND  (56 unrouted)
  Top 0.406: IC11.10 111.76,61.59 111.76,55.88 IC12.7
  pour Bottom (isolate 0.61): 0,100.01 160.02,100.01 160.02,89.53 160.02,0 0,0
  pour Top (isolate 0.61): 0,100.01 160.02,100.01 160.02,97.16 160.02,0 0,0
IRQ0
  Top 0.406: JP1.2 RN1.9
  Bottom 0.406: JP1.2 129.86,97.79 91.12,97.79 78.74,85.41 IC5.18
IRQ1
  Top 0.406: JP1.4 RN1.8
  Bottom 0.406: JP1.4 141.92,83.19 139.38,83.19 125.73,96.84 92.71,96.84 81.28,85.41 IC5.17
IRQ2
  Top 0.406: RN1.7 JP1.6
  Bottom 0.406: JP1.6 141.92,80.64 139.38,80.64 124.14,95.89 99.38,95.89 88.9,85.41 IC5.14
IRQ3
  Top 0.406: JP1.8 RN1.6
  Bottom 0.406: JP1.8 141.92,78.11 139.38,78.11 122.56,94.93 100.97,94.93 91.44,85.41 IC5.13
IRQ4
  Top 0.406: JP1.10 RN1.5
  Bottom 0.406: JP1.10 141.92,75.56 139.38,75.56 120.97,93.98 107.63,93.98 98.42,84.77 98.42,75.56 97.47,74.61 93.98,74.61 91.44,77.15 IC5.8
IRQ5
  Top 0.406: JP1.12 RN1.4
  Bottom 0.406: JP1.12 141.92,73.03 139.38,73.03 121.6,90.81 105.73,90.81 99.38,84.45 99.38,75.25 97.79,73.66 92.39,73.66 88.9,77.15 IC5.7
IRQ6
  Top 0.406: JP1.14 RN1.3
  Bottom 0.406: JP1.14 141.92,70.48 139.38,70.48 120.02,89.85 106.05,89.85 100.33,84.14 100.33,74.93 98.11,72.71 85.72,72.71 81.28,77.15 IC5.4
IRQ7
  Top 0.406: JP1.16 RN1.2
  Bottom 0.406: JP1.16 141.92,67.94 139.38,67.94 120.33,87 104.46,87 101.28,83.82 101.28,74.61 98.42,71.75 84.14,71.75 78.74,77.15 IC5.3
N$1
  Top 0.406: IC6.9 43.5,54.29 IC8.1
N$2
  Top 0.406: IC2.15 19.05,59.05 22.23,55.88 28.26,55.88 30.48,53.66 30.48,45.72 IC3.10
  Bottom 0.406: IC3.7 IC3.10
N$3  (via drill 0.61 pad 1.27)
  Top 0.406: IC8.2 46.99,50.8 v46.99,48.26
  Bottom 0.406: v46.99,48.26 60.33,48.26 63.5,45.09 IC7.9
N$4
  Top 0.406: IC6.7 44.77,83.82 44.77,69.53 49.53,64.77 49.53,56.83 53.34,53.02 IC8.4
N$5
  Top 0.406: IC8.5 57.15,50.8 57.15,41.59 60.96,37.78 IC7.7
N$6
  Top 0.406: IC8.10 54.61,58.42 54.61,41.59 58.42,37.78 IC7.6
N$7
  Top 0.406: IC6.6 47.31,83.82 47.31,72.39 58.42,61.28 IC8.9
N$9  (via drill 0.61 pad 1.27)
  Top 0.406: IC10.11 86.36,60.64 80.96,66.04 v56.83,66.04 56.83,76.83 IC6.14 | IC8.12 v50.8,66.04
  Bottom 0.406: v50.8,66.04 v56.83,66.04
N$10  (via drill 0.61 pad 1.27)
  Top 0.406: IC8.13 48.26,55.24 49.53,53.98 49.53,45.72 IC7.14 | v113.03,39.05 120.65,31.43 120.65,24.77 121.92,23.5 IC4.12
  Bottom 0.406: IC7.14 50.8,43.81 53.02,41.59 70.17,41.59 72.71,39.05 v113.03,39.05
N$11
  Bottom 0.406: IC10.14 78.74,59.05 76.2,56.52 72.07,56.52 70.8,55.24 59.37,55.24 58.42,54.29 52.39,54.29 50.8,52.7 IC8.3
N$12
  Bottom 0.406: IC10.13 81.28,59.05 77.79,55.56 72.39,55.56 71.12,54.29 59.69,54.29 58.42,53.02 IC8.6
N$13
  Top 0.406: IC8.8 60.96,61.91 63.5,64.45 81.28,64.45 83.82,61.91 IC10.12
N$14  (via drill 0.61 pad 1.27)
  Top 0.406: v53.34,64.14 IC8.11 | IC12.2 101.6,53.34 101.6,61.91 99.38,64.14 v97.47,64.14
  Bottom 0.406: v97.47,64.14 v53.34,64.14
N$16
  Bottom 0.406: IC11.5 111.76,74.3 122.87,74.3 128.27,68.9 128.27,58.42 132.08,54.61 134.62,54.61 135.89,53.34 135.89,49.85 137.16,48.58 139.7,48.58 140.97,47.31 140.97,39.37 IC13.6
N$18
  Bottom 0.406: IC10.3 78.74,52.39 80.64,54.29 81.92,54.29 82.55,53.66 82.55,50.16 91.44,41.27 118.43,41.27 124.46,35.24 127.32,35.24 129.54,37.47 IC13.2
N$19
  Bottom 0.406: IC10.4 81.28,50.16 91.12,40.32 118.11,40.32 124.14,34.29 133.67,34.29 137.16,37.78 IC13.5
N$20
  Bottom 0.406: IC13.11 136.21,42.23 91.76,42.23 83.82,50.16 IC10.5
N$21
  Bottom 0.406: IC13.14 129.54,43.18 92.08,43.18 86.36,48.9 IC10.6
N$22
  Bottom 0.406: IC14.13 134.62,70.17 119.06,85.72 IC11.19
N$23
  Bottom 0.406: IC11.16 124.14,78.11 133.35,68.9 133.35,58.1 134.3,57.15 140.34,57.15 142.24,59.05 IC14.10
N$24
  Bottom 0.406: IC11.15 124.14,75.56 130.81,68.9 130.81,58.1 133.03,55.88 136.21,55.88 139.7,52.39 IC14.6
N$25
  Bottom 0.406: IC11.12 118.75,67.94 125.73,60.96 125.73,58.42 IC14.3
N$26
  Top 0.406: IC11.2 102.87,80.64 102.87,67.31 109.22,60.96 109.22,50.48 124.46,35.24 130.18,35.24 132.08,37.15 IC13.3
N$27
  Top 0.406: IC6.5 51.12,86.36 49.21,88.27 42.86,88.27 38.1,83.5 38.1,20.95 43.18,15.88 95.89,15.88 97.79,17.78 IC9.6
N$28  (via drill 0.61 pad 1.27)
  Top 0.406: IC13.10 142.24,45.09 138.11,40.96 134.62,40.96 133.35,39.69 133.35,35.56 132.08,34.29 121.6,34.29 106.68,49.21 106.68,53.98 104.14,56.52 104.14,62.55 99.38,67.31 v99.38,68.9
  Bottom 0.406: v99.38,68.9 106.05,75.56 IC11.6
N$30
  Bottom 0.406: IC11.9 109.22,66.67 118.75,66.67 124.78,60.64 124.78,50.16 127.32,47.62 132.72,47.62 IC13.13
N$47
  Top 0.406: IC12.5 113.35,49.21 124.14,49.21 IC14.1 128.27,50.8 128.27,39.37 IC13.1
N$57
  Bottom 0.406: IC6.4 53.66,85.41 56.83,88.58 74.3,88.58 76.2,86.68 IC5.19
N$58
  Bottom 0.406: IC6.3 58.74,87.63 73.98,87.63 74.93,86.68 74.93,83.5 75.88,82.55 81.92,82.55 83.82,84.45 IC5.16
N$59
  Bottom 0.406: IC5.15 86.36,84.45 83.5,81.6 73.34,81.6 72.39,82.55 61.28,82.55 IC6.2
N$60
  Top 0.406: IC5.12 91.44,82.55 63.82,82.55 IC6.1
N$61
  Top 0.406: IC5.9 89.85,81.6 56.2,81.6 53.66,79.06 IC6.13
N$62
  Top 0.406: IC6.12 51.12,76.83 52.7,75.25 54.29,75.25 54.93,75.88 54.93,79.06 56.52,80.64 83.82,80.64 86.36,78.11 IC5.6
N$63
  Bottom 0.406: IC5.5 83.82,78.11 82.23,79.69 75.56,79.69 74.93,79.06 74.93,75.88 73.98,74.93 50.48,74.93 48.58,76.83 IC6.11
N$64
  Bottom 0.406: IC5.2 76.2,75.88 74.3,73.98 48.9,73.98 46.04,76.83 IC6.10
OP0
  Top 0.406: JP7.9 149.54,35.88 136.53,35.88 134.62,37.78 IC13.4
OP1
  Top 0.406: JP7.8 146.05,42.23 142.24,38.42 IC13.7
OP2
  Top 0.406: JP7.7 145.73,44.77 IC13.9
OP3
  Top 0.406: JP7.6 152.08,47.31 151.45,47.94 139.38,47.94 IC13.12
OP4
  Top 0.406: JP7.5 136.84,49.85 IC14.4
OP5
  Top 0.406: JP7.4 152.08,52.39 150.18,54.29 144.46,54.29 IC14.7
OP6
  Top 0.406: JP7.3 152.08,54.93 147.32,59.69 IC14.9
OP7
  Top 0.406: JP7.2 150.81,57.47 146.37,61.91 139.38,61.91 IC14.12
OP8
  Top 0.406: JP7.1 149.54,60.01 146.69,62.87 123.83,62.87 117.47,56.52 117.47,51.12 116.52,50.16 114.62,50.16 113.03,51.75 IC12.6
PROT
  Top 0.406: IC4.10 116.84,18.41 108.9,10.48 103.82,10.48 JP10.21
RST  (via drill 0.61 pad 1.27)
  Top 0.406: IC10.15 77.47,58.42 77.47,44.45 v85.41,36.51 | v97.16,36.51 v107.95,25.72
  Bottom 0.406: v85.41,36.51 v97.16,36.51 | v107.95,25.72 107.95,17.14 JP10.9

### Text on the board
Top: #1
_tsilk: VCC2 | GND1 | IC11 | 74LS273N | JP3 | JP1 | IC6 | 74LS148N | 74LS273N | IC5 | JP8 | RN1 | 1 | JP7 | 74LS163 | 74LS08N | 74LS173N | 74LS74N | 74LS157N | IC10 | IC2 | IC8 | IC12 | IC14 | 74LS157N | 74LS163 | 74LS148N | IC13 | IC3 | IC7 | JP4 | JP2 | IC1 | IC4 | 74LS08N | 74LS00N | 74S32N | IC9 | GND2 | VCC1 | JP10 | 10u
